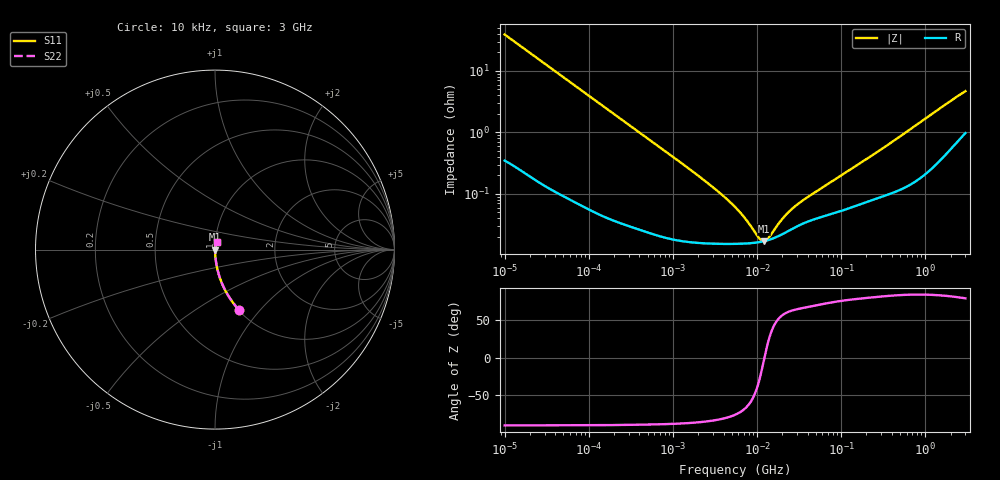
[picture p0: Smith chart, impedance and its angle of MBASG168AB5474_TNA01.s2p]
! MBASG168AB5474_TNA01  S-PARAMETER MODEL  ( Standard Model )
! Model Generated by TAIYO YUDEN Corporation (http://www.ty-top.com)
! Version 1.0
! TAIYO YUDEN Control No. 220601
! Copyright(c) 2012 TAIYO YUDEN CO.,LTD. All Rights Reserved.
! Product Description (link to TY-COMPAS)
! https://ds.yuden.co.jp/TYCOMPAS/or/detail?pn=MBASG168AB5474KTNA01&u=M
! Products Name : Multilayer Ceramic Capacitors
! Characteristics :
!  Capacitance : 0.47 [uF] , Rated Voltage : 35 [V] , TCC : X5R
!  Case Size : 1.6 x 0.8 / 0.063 x 0.031 [mm/inch] , Thickness : 0.8 / 0.031 [mm/inch]
!  (Conditions: Temperature = 25 [degC] , DC Bias Voltage = 0 [V])
! External Node Assignments :
!  1  o---| |---o  2
! GND o---------o GND
! Frequency Range : 10kHz  -  3GHz  [ 401 STEP ]
# MHZ S RI R 50
! Freq[MHz].  S11 Real  S11 Imag  S21 Real  S21 Imag  S12 Real  S12 Imag  S22 Real  S22 Imag
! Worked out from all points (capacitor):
!   401 points, 10 kHz to 3 GHz, reference 50 ohm
!   read as one part in series: C = 405 nF near 10.65 kHz
!   lowest |Z| = 17.1 mohm at 12.05 MHz (marker M1)
!   series resonance near 12.27 MHz, so ESL is about 410 pH
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0.01  0.1354 -0.3377  0.8646 0.3377  0.8646 0.3377  0.1354 -0.3377
0.016047  0.0586 -0.2301  0.9414 0.2301  0.9414 0.2301  0.0586 -0.2301
0.027426  0.0216 -0.1405  0.9784 0.1405  0.9784 0.1405  0.0216 -0.1405
0.045421  0.00849 -0.0863  0.9915 0.0863  0.9915 0.0863  0.00849 -0.0863
0.082683  0.00294 -0.0479  0.9971 0.0479  0.9971 0.0479  0.00294 -0.0479
0.683653  0.000242 -0.00589  0.9998 0.00589  0.9998 0.00589  0.000242 -0.00589
2.652321  0.000158 -0.00146  0.9998 0.00146  0.9998 0.00146  0.000158 -0.00146
3.996065  0.000155 -0.00091  0.9998 0.00091  0.9998 0.00091  0.000155 -0.00091
5.477226  0.000155 -0.000596  0.9998 0.000596  0.9998 0.000596  0.000155 -0.000596
7.274378  0.000156 -0.000364  0.9998 0.000364  0.9998 0.000364  0.000156 -0.000364
10.61963  0.000165 -9.66e-05  0.9998 9.66e-05  0.9998 9.66e-05  0.000165 -9.66e-05
11.31085  0.000167 -5.43e-05  0.9998 5.43e-05  0.9998 5.43e-05  0.000167 -5.43e-05
12.04705  0.00017 -1.23e-05  0.9998 1.23e-05  0.9998 1.23e-05  0.00017 -1.23e-05
12.83117  0.000174 2.95e-05  0.9998 -2.95e-05  0.9998 -2.95e-05  0.000174 2.95e-05
13.66633  0.000178 7.13e-05  0.9998 -7.13e-05  0.9998 -7.13e-05  0.000178 7.13e-05
18.73182  0.000212 0.000281  0.9998 -0.000281  0.9998 -0.000281  0.000212 0.000281
24.10585  0.000254 0.000451  0.9997 -0.000451  0.9997 -0.000451  0.000254 0.000451
31.02164  0.000305 0.000625  0.9997 -0.000625  0.9997 -0.000625  0.000305 0.000625
45.28751  0.000378 0.000918  0.9996 -0.000918  0.9996 -0.000918  0.000378 0.000918
374.4521  0.00103 0.00645  0.999 -0.00645  0.999 -0.00645  0.00103 0.00645
1811.492  0.00541 0.029  0.9946 -0.029  0.9946 -0.029  0.00541 0.029
3000  0.0117 0.045  0.9883 -0.045  0.9883 -0.045  0.0117 0.045
